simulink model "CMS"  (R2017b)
settings: Solver=FixedStepDiscrete  StartTime=0.0  StopTime=10.0  FixedStep=0.01  RelTol=1e-3  EnableMultiTasking=on
undefined symbols (not defined in the file): ASWTYPE_FALSE, ASWTYPE_TRUE, CcCMS_CANSendDelay_ms, CcCMS_ChrgMaxPackVoltLimt_V, CcCMS_PeakVoltCh_V, CcCMS_PeakVoltDisCh_V, CcSOC_DispSOCHighThrhd_pct, CMS09D_RUNTIME_MS, CMS_CONST0_NUMB, CMS_CONST1000_NUMB, CMS_CONST100_NUMB, CMS_CONST1_NUMB, CMS_CONST2047_NUMB, CMS_CONST2_NUMB, CMS_CONST3_NUMB, CMS_CONST4_NUMB, CMS_CONST5_NUMB, CMS_CONST6_NUMB, CMS_CONST7_NUMB, CMS_CONSTF1_NUMB, Enum_ACCACChrgState, Enum_CMSACChgMode, Enum_CMSBmsSelfChk, Enum_CMSBmsSt, Enum_CMSChgMode, Enum_CMSDCChgMode, Enum_CMSHVBatFltSevrtyStat, Enum_CMSHVConnSt, Enum_CMSPreThmMode, Enum_CMSPreThmReq, Enum_CMSThmPropagation, Enum_CTCCtrCtlConnMode, Enum_CTCCtrCtlState, Enum_DCCDCChrgState, Enum_DCCDCConnSt, Enum_ISOHVIsoFltLevel, Enum_MSMBMUState, Enum_ODPCCState, Enum_VDPPreThmEna
libraries: AIWAYS_Powertrain_BMS_lib x148
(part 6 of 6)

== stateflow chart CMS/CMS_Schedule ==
  (default) -> (junction 50)
  (junction 50) -> (junction 13) : { CMS_09D_10ms; }
  (junction 13) -> (junction 150) : { TimeCounter20ms ++; TimeCounter100ms ++; TimeCounter500ms ++; TimeCounter1000ms ++; }
  (junction 150) -> (junction 422) : [TimeCounter20ms >= Const20ms]
  (junction 150) -> (junction 424)
  (junction 422) -> (junction 424) : { CMS_3E0_20ms; TimeCounter20ms = 0; }
  (junction 424) -> (junction 503) : [TimeCounter100ms >= Const100ms]
  (junction 424) -> (junction 505)
  (junction 503) -> (junction 505) : {CMS_2C0_100ms; CMS_2C2_100ms; CMS_2C3_100ms; CMS_2C7_100ms; CMS_2C8_100ms; CMS_2CA_100ms; CMS_2CD_100ms; CMS_2CE_100ms; CMS_2CF_100ms; CMS_3E1_100ms; TimeCounter100ms = 0; }
  (junction 505) -> (junction 509) : [TimeCounter500ms >= Const500ms]
  (junction 505) -> (junction 512)
  (junction 509) -> (junction 512) : {CMS_318_500ms; TimeCounter500ms = 0; }
  (junction 512) -> (junction 533) : [TimeCounter1000ms >= Const1000ms]
  (junction 512) -> (junction 536)
  (junction 533) -> (junction 536) : {CMS_3B0_1000ms; TimeCounter1000ms = 0; }
  data: TimeCounter20ms local uint8; Const100ms constant uint8 =10; TimeCounter100ms local uint8; Const20ms constant uint8 =2; Const500ms constant uint8 =50; TimeCounter500ms local uint8; TimeCounter1000ms local uint8; Const1000ms constant uint8 =100
  events: output FUNCTION_CALL_EVENT; output FUNCTION_CALL_EVENT; output FUNCTION_CALL_EVENT; output FUNCTION_CALL_EVENT; output FUNCTION_CALL_EVENT; output FUNCTION_CALL_EVENT; output FUNCTION_CALL_EVENT; output FUNCTION_CALL_EVENT; output FUNCTION_CALL_EVENT; output FUNCTION_CALL_EVENT; output FUNCTION_CALL_EVENT; output FUNCTION_CALL_EVENT; output FUNCTION_CALL_EVENT; output FUNCTION_CALL_EVENT
